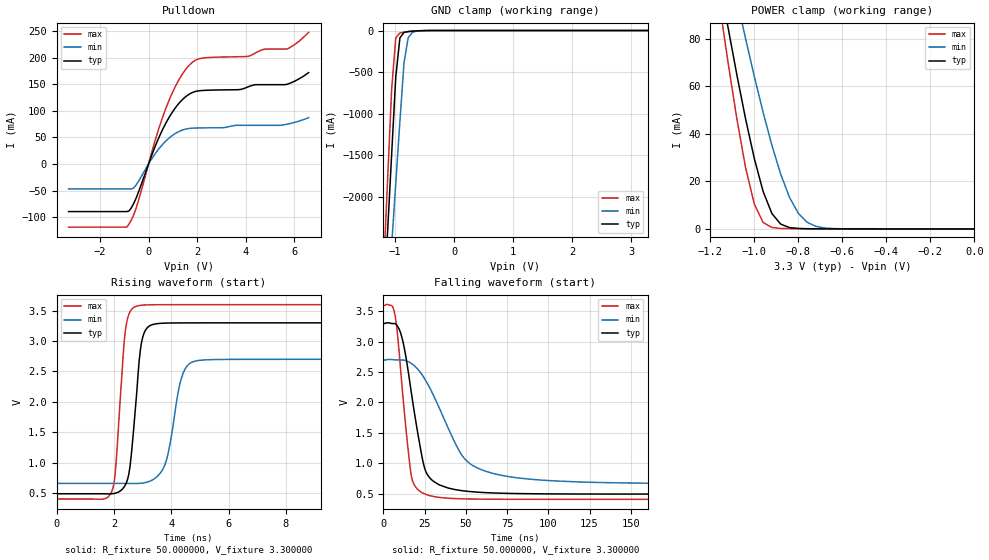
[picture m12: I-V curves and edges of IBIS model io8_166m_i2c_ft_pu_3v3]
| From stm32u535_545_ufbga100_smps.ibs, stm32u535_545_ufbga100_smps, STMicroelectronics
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|   Model io8_166m_i2c_ft_pu_3v3
[Model]  io8_166m_i2c_ft_pu_3v3
Model_type I/O_open_drain
Polarity   Non-Inverting
Enable   Active-Low
Vinl =   0.990000V
Vinh =   2.310000V
Vmeas =  1.650000V
Cref =   50.000000pF
Rref =   100.000000M
Vref =   1.650000V
C_comp   3.523800pF   3.496000pF   3.564000pF
[Temperature Range]   25.000000   0.140000k   -40.000000
[Pullup Reference]   3.300000V   2.700000V   3.600000V
[Pulldown Reference]   0.0V   0.0V   0.0V
[POWER Clamp Reference]   3.300000V   2.700000V   3.600000V
[GND Clamp Reference]   0.0V   0.0V   0.0V
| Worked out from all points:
|   slope of the pulldown table from 0 to 0.495 V, typ, clamps not added: 8.73 ohm
|   GND clamp passes 1 mA (typ) near -0.50 V on its own axis
|   POWER clamp passes 1 mA (typ) near -0.85 V on its own axis
|   rising waveform, R_fixture 50.000000, V_fixture 3.300000: 20-80 % time 307ps typ, 454ps min, 272ps max; typ from 0.49 V to 3.3 V
|   falling waveform, R_fixture 50.000000, V_fixture 3.300000: 20-80 % time 10.1ns typ, 22.3ns min, 6.6ns max; typ from 3.3 V to 0.49 V
[Pulldown]
|Voltage   I(typ)   I(min)   I(max)
-3.3V     -89.71mA   -47.06mA   -119mA
-900mV    -89.71mA   -47.06mA   -119mA
-500mV    -62.92mA   -38.72mA   -81.44mA
300mV     36.2mA     21.01mA    48.7mA
800mV     84.07mA    46.96mA    114.8mA
1.3V      116.7mA    62.09mA    162.4mA
1.8V      134.4mA    67.39mA    191.2mA
2.3V      138.6mA    67.98mA    199.8mA
4.1V      145.2mA    72.76mA    202.7mA
4.8V      149.3mA    72.76mA    216.4mA
5.7V      149.8mA    74.9mA     216.4mA
6.6V      172mA      87.1mA     247.9mA
[GND_clamp]
|Voltage   I(typ)   I(min)   I(max)
-3.3V     -9.098A    -9.372A    -9.671A
-1.2V     -3.386A    -4.091A    -2.933A
-1.13V    -2.437A    -3.34A     -1.815A
-1.06V    -1.49A     -2.588A    -705.6mA
-990mV    -555.7mA   -1.839A    -89.03mA
-920mV    -88.12mA   -1.093A    -28.78mA
-850mV    -22.35mA   -387.4mA   -19.84mA
-780mV    -12.12mA   -88.01mA   -13.88mA
-710mV    -7.71mA    -22.52mA   -8.846mA
-640mV    -4.545mA   -7.864mA   -4.87mA
-360mV    -31.12uA   -173.5uA   -8.497uA
3.28V     0A         14.15nA    -7.901nA
[POWER_clamp]
|Voltage   I(typ)   I(min)   I(max)
-3.28V    1.355A     1.167A     1.665A
-1.16V    105.8mA    131.6mA    95.87mA
-1.12V    85.08mA    114mA      70.45mA
-1.08V    65.17mA    96.88mA    46.74mA
-1.04V    46.48mA    80.2mA     25.96mA
-1V       29.63mA    64.18mA    10.49mA
-960mV    15.81mA    49.06mA    2.743mA
-920mV    6.481mA    35.16mA    612.1uA
-840mV    577.5uA    13.29mA    137.7uA
-760mV    93.73uA    2.807mA    97.78uA
-640mV    40.06uA    158.9uA    59.33uA
0V        0A         19.33nA    0A
[Ramp]
| variable   typ   min   max
dV/dt_r  1.68571/0.50351n   1.22376/0.57492n   1.91753/0.30421n
dV/dt_f  1.68571/10.06838n   1.22376/22.26885n   1.91753/6.56998n
R_load = 50.000000
[Rising Waveform]
R_fixture= 50.000000
V_fixture= 3.300000
V_fixture_min= 2.700000
V_fixture_max= 3.600000
|time   V(typ)   V(min)   V(max)
0s        490.5mV    660.4mV    404.1mV
1.922ns   490.2mV    660.4mV    524.4mV
2.042ns   499mV      660.4mV    806.8mV
2.402ns   640.4mV    660.1mV    3.18V
2.763ns   1.96V      659.2mV    3.568V
3.123ns   3.194V     677mV      3.593V
3.764ns   3.294V     947.9mV    3.597V
4.364ns   3.297V     2.403V     3.597V
4.845ns   3.298V     2.671V     3.597V
19.94ns   3.3V       2.7V       3.6V
[Falling Waveform]
R_fixture= 50.000000
V_fixture= 3.300000
V_fixture_min= 2.700000
V_fixture_max= 3.600000
|time   V(typ)   V(min)   V(max)
0s        3.3V       2.7V       3.6V
5.606ns   3.3V       2.707V     3.583V
7.207ns   3.299V     2.701V     3.417V
12.01ns   2.983V     2.699V     2.046V
17.62ns   2.039V     2.631V     712.3mV
24.02ns   1.023V     2.433V     506.5mV
27.23ns   791.1mV    2.286V     471.7mV
49.65ns   540.3mV    1.061V     411.2mV
76.08ns   501.9mV    778.4mV    405mV
398.8ns   490.5mV    660.4mV    404.1mV
